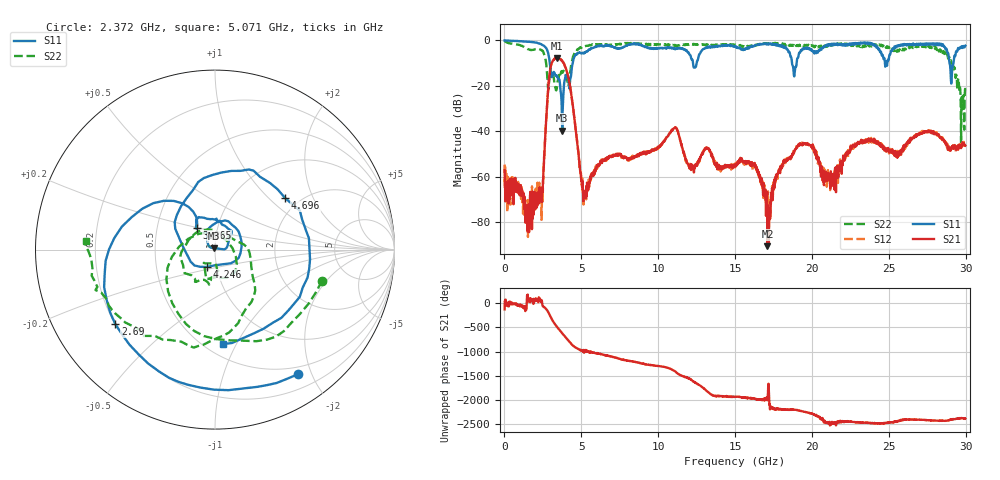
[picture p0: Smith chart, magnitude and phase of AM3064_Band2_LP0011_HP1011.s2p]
# Hz S DB R 50.0
!freq dBS11 angS11 dBS21 angS21 dBS12 angS12 dBS22 angS22
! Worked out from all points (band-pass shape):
!   1600 points, 10 MHz to 29.98 GHz, reference 50 ohm
!   highest |S21| = -7.71 dB at 3.403 GHz (marker M1); lowest = -90.4 dB at 17.1 GHz (marker M2)
!   |S21| within 3 dB of the highest: 3.037 GHz to 3.896 GHz (859.8 MHz wide, 24.8 % of centre)
!   lowest |S11| = -39.6 dB at 3.759 GHz (marker M3), VSWR 1.02, Z = 49.2 + j0.68 ohm
!   |S11| at or under -10 dB: 2.953 GHz to 4.442 GHz (1.489 GHz wide, 40.3 % of centre); 18.71 GHz to 19.01 GHz (298.6 MHz wide, 1.58 % of centre); 28.95 GHz to 29.2 GHz (254.4 MHz wide, 0.875 % of centre)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
!   |S22| runs from -45.7 to -0.2 dB; largest |S21 - S12| = 0.014
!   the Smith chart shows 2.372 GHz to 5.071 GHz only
!   S11 on the Smith chart (normalised r, x): 2.372 GHz: 0.39, -1.79; 2.69 GHz: 0.20, -0.32; 3.065 GHz: 0.79, +0.20; 4.246 GHz: 0.90, -0.18; 4.696 GHz: 1.70, +1.27; 5.071 GHz: 0.60, -0.88
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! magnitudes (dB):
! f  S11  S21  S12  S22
! 10 MHz  0.0  -57.0  -54.6  -0.2
! 1.491 GHz  -0.6  -77.9  -79.7  -3.8
! 2.372 GHz  -1.6  -69.2  -69.4  -4.1
! 2.69 GHz  -3.2  -37.7  -37.7  -9.1
! 3.065 GHz  -16.0  -10.1  -10.0  -16.3
! 3.403 GHz  -15.6  -7.7  -7.8  -21.3
! 3.759 GHz  -39.6  -9.0  -9.1  -14.1
! 4.246 GHz  -19.4  -19.3  -19.4  -14.8
! 4.696 GHz  -6.3  -42.7  -42.7  -4.6
! 5.015 GHz  -5.8  -61.6  -61.9  -3.2
! 5.071 GHz  -5.5  -61.8  -66.0  -2.9
! 10 GHz  -3.5  -46.9  -47.6  -1.8
! 11.11 GHz  -3.9  -38.3  -38.3  -2.3
! 15 GHz  -2.7  -55.5  -55.8  -1.9
! 16.28 GHz  -2.2  -53.8  -55.0  -2.2
! 17.1 GHz  -1.5  -90.4  -77.6  -1.3
! 19.99 GHz  -4.2  -46.6  -46.7  -2.1
! 21.27 GHz  -1.5  -59.1  -61.8  -2.0
! 23.08 GHz  -1.4  -45.3  -44.8  -2.1
! 25 GHz  -8.4  -48.2  -48.9  -2.8
! 28.56 GHz  -2.5  -43.5  -43.2  -4.7
! 29.98 GHz  -2.4  -46.2  -45.8  -21.6
